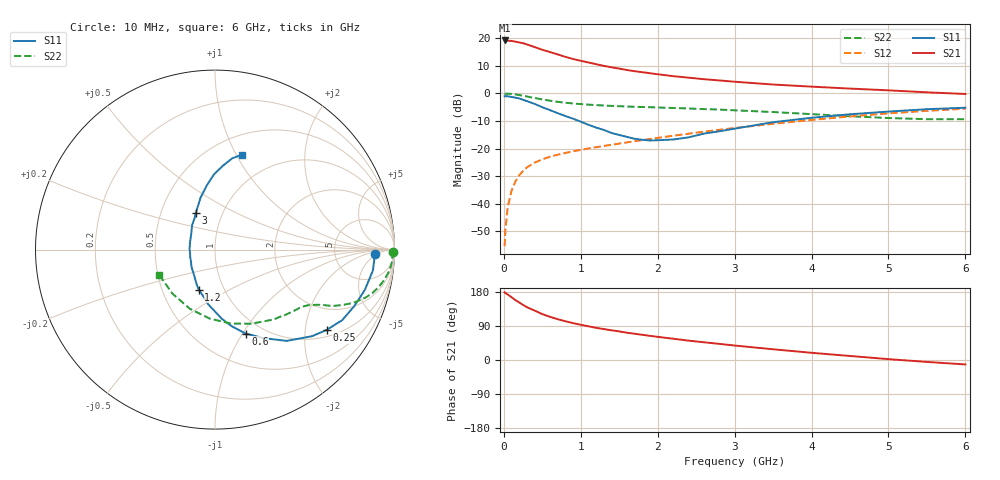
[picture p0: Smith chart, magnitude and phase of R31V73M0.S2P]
! SIEMENS Small Signal Semiconductors
! BFR181
! Si NPN RF Bipolar Junction Transistor in SOT23
! VCE = 1.75 V  IC = 3 mA
! Common Emitter S-Parameters:  May  1996
# GHz  S  MA  R  50
!  f  S11  S21  S12  S22
! GHz  MAG  ANG  MAG  ANG  MAG  ANG  MAG  ANG
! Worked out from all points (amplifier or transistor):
!   36 points, 10 MHz to 6 GHz, reference 50 ohm
!   highest |S21| = 19.2 dB at 10 MHz (marker M1)
!   |S21| within 3 dB of that: start of sweep to 461.6 MHz
!   unconditionally stable (mu >= 1): 1.327 GHz to 3.23 GHz
!   at 250 MHz: K = 0.31, MSG = 23.1 dB, |S12| = -28.1 dB
!   at 1.4 GHz: K = 1.02, MAG = 13.1 dB, |S12| = -18.6 dB
!   at 6 GHz: K = 0.87, MSG = 2.7 dB, |S12| = -5.5 dB
!   S11 on the Smith chart (normalised r, x): 10 MHz: 16, -4; 250 MHz: 1.20, -2.61; 600 MHz: 0.83, -1.03; 1.2 GHz: 0.76, -0.36; 3 GHz: 0.75, +0.32; 6 GHz: 0.70, +1.06
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0.01  0.8894 -1.6  9.133 178.7  0.0017 92.8  0.9945 -0.7
0.02  0.89 -2.9  9.112 177.0  0.0033 87.5  0.9872 -1.4
0.05  0.8876 -7.5  9.03 172.8  0.0086 85.1  0.9902 -3.5
0.1  0.8644 -15.1  8.953 165.8  0.0172 82.0  0.9792 -6.8
0.15  0.8375 -22.1  8.688 158.1  0.0253 77.3  0.9578 -10.2
0.25  0.7664 -35.7  8.135 145.3  0.0394 70.5  0.9092 -15.5
0.3  0.7251 -41.7  7.747 139.4  0.0456 68.5  0.8799 -17.7
0.4  0.6463 -51.9  6.928 130.4  0.0556 64.2  0.8272 -21.0
0.5  0.5622 -61.3  6.193 121.1  0.0638 61.3  0.7787 -23.3
0.6  0.4979 -70.0  5.629 113.9  0.0713 58.9  0.7378 -25.1
0.7  0.4381 -77.5  5.103 107.7  0.0773 58.4  0.7047 -26.3
0.8  0.3892 -84.1  4.609 102.2  0.0833 57.6  0.678 -27.1
0.9  0.3483 -89.5  4.211 97.3  0.0894 57.1  0.6575 -27.9
1.1  0.2701 -103.7  3.642 88.9  0.1005 57.3  0.6265 -29.5
1.2  0.2401 -112.2  3.391 84.9  0.1059 57.6  0.614 -30.2
1.6  0.1628 -143.6  2.66 72.0  0.1295 58.7  0.5792 -33.5
2.2  0.1461 161.4  2.056 56.2  0.1709 58.9  0.5446 -40.4
3  0.2298 117.8  1.63 38.2  0.236 56.2  0.4944 -53.0
3.5  0.3008 105.5  1.45 28.3  0.2819 52.9  0.4599 -63.9
4.5  0.4191 90.8  1.224 10.6  0.383 43.4  0.3854 -94.5
5.5  0.5176 79.3  1.048 -5.1  0.4837 30.7  0.3411 -134.2
6  0.5506 74.0  0.977 -11.7  0.5292 23.5  0.3409 -155.6
